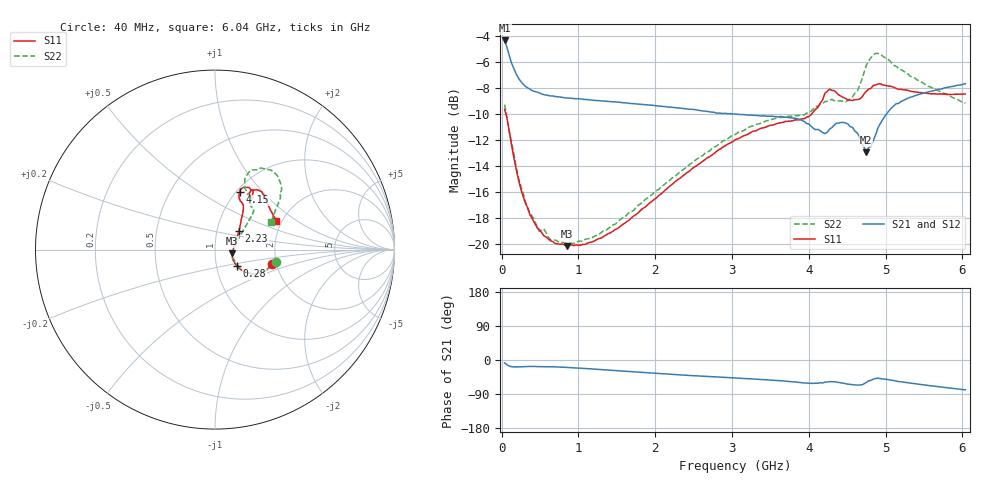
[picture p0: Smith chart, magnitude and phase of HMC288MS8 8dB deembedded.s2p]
!Hittite Microwave Corporation
!12 Elizabeth Drive
!Chelmsford, MA 01824
!Tel: 978-250-3343
!Fax: 978-250-3373
!Device: HMC288MS8, 0.7-3.7 GHz GaAs IC 3-bit Digital Attenuator in 8-lead Grounded Base surface Mount Plastic Package
!Misc:  8dB state, room
# GHZ S DB R 50.0
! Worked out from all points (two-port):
!   201 points, 40 MHz to 6.04 GHz, reference 50 ohm
!   highest |S21| = -4.33 dB at 40 MHz (marker M1); lowest = -12.9 dB at 4.75 GHz (marker M2)
!   |S21| within 3 dB of the highest: start of sweep to 232.7 MHz
!   lowest |S11| = -20.2 dB at 850 MHz (marker M3), VSWR 1.22, Z = 60.6 - j2.5 ohm
!   |S11| at or under -10 dB: 57.09 MHz to 4.036 GHz (3.979 GHz wide, 194 % of centre)
!   |S22| runs from -20.0 to -5.3 dB; largest |S21 - S12| = 0.0044
!   S11 on the Smith chart (normalised r, x): 40 MHz: 1.90, -0.35; 280 MHz: 1.25, -0.24; 2.23 GHz: 1.28, +0.28; 4.15 GHz: 1.04, +0.76; 6.04 GHz: 1.87, +0.70
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0.04  -9.62 -14.5  -4.33 -7.7  -4.39 -7.6  -9.27 -11.2
0.07  -10.29 -22.9  -4.85 -12.7  -4.86 -12.7  -10.23 -21.4
0.13  -12.37 -33.8  -6.06 -17.6  -6.01 -17.2  -12.19 -33.3
0.28  -16.30 -36.9  -7.69 -17.3  -7.64 -17.7  -16.06 -34.6
0.49  -18.87 -28.1  -8.36 -17.4  -8.37 -17.4  -19.02 -26.8
0.85  -20.16 -12.0  -8.76 -19.6  -8.76 -19.8  -19.94 -9.1
1.06  -20.02 -2.8  -8.86 -22.1  -8.88 -22.2  -19.79 0.2
1.51  -18.80 15.9  -9.08 -28.3  -9.08 -28.4  -18.29 15.9
2.05  -16.23 33.9  -9.38 -35.6  -9.38 -35.8  -15.78 29.8
2.23  -15.37 38.3  -9.48 -38.0  -9.48 -38.1  -14.87 32.7
3.04  -11.98 52.3  -10.01 -47.4  -9.96 -47.6  -11.58 41.6
3.82  -10.45 59.4  -10.32 -57.9  -10.32 -57.9  -10.11 47.5
4.06  -9.83 65.5  -11.09 -61.5  -11.04 -61.7  -9.60 53.5
4.15  -9.15 66.3  -11.28 -60.1  -11.29 -60.3  -9.23 53.8
4.27  -8.08 61.1  -11.16 -57.0  -11.13 -57.0  -8.96 53.6
4.51  -8.91 55.8  -10.76 -63.8  -10.76 -63.8  -8.97 59.1
4.63  -8.89 57.4  -11.43 -66.0  -11.43 -66.0  -8.26 64.3
4.75  -8.25 58.9  -12.92 -59.2  -12.87 -59.7  -6.26 65.7
4.9  -7.69 52.3  -11.08 -48.0  -11.10 -48.5  -5.33 51.6
5.05  -7.86 47.0  -9.71 -52.4  -9.68 -52.3  -5.87 43.2
5.32  -8.24 40.6  -8.71 -61.1  -8.67 -61.1  -7.07 36.8
6.04  -8.45 25.3  -7.66 -78.8  -7.66 -78.7  -9.16 25.8
